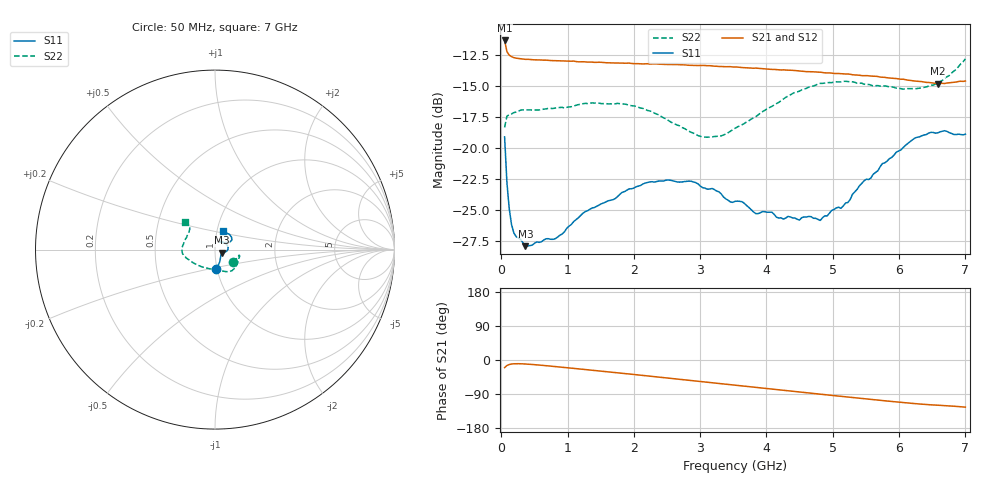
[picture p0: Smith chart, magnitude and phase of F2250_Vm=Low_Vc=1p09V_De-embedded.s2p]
! Integrated Device Technology
! Corporate Headquarters
! 6024 Silver Creek Valley Road
! San Jose, CA 95138  USA
! Phone:  1-408-284-8200
! Toll Free:  1-800-223-1366
! Webpage:  http://www.idt.com/
! Timing and RF Division
! 515 Groton Road, Suite 102
! Westford, MA 01886-6024
! Device:  F2250
! Description: Voltage Variable RF Attenuator
! Frequency:  50.0 -  6000.00 MHz
! Package:  3x3 mm Thin QFN Plastic Package: 16 pin
! Ports:  2 RF, 3 DC
!  Pin  1  = GND
!  Pin  2  = NC
!  Pin  3  = RF1  = Port 1
!  Pin  4  = NC
!  Pin  5  = GND
!  Pin  6  = GND
!  Pin  7  = GND
!  Pin  8  = GND
!  Pin  9  = NC
!  Pin 10  = RF2  = Port 2
!  Pin 11  = NC
!  Pin 12  = GND
!  Pin 13  = GND
!  Pin 14  = VCNTRL
!  Pin 15  = VDD
!  Pin 16  = VMODE
! Vcntrl:  1.090 Volts
! Vmode:  +0.000 Volts
! Vdd:  +3.30  Volts
! Current:  1.191 mA
! Data:  The device was measured on a the F2250 evaluation board which has
!  individual transmission lines to the RF pins.  Data was collected
!  using a calibrated network analyzer.  The evaluation board was
!  de-embedded using a TRL calibration technique.
!  The reference plane is the edge of the package pin.
! Misc:  SN 10
!  Action Tracker AT0258
! Date Measured:  2014-11-26
! Date:  2015-10-15  MJV
! Note:
!  Integrated Device Technology supplies this data as a sample of measured
!  data at the package pin for this product.  Your particular data for this
!  product may vary.
!  Data was taken at 25 degrees C.
!  Integrated Device Technology reserves the right to change this data at anytime.
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# GHz S dB R 50
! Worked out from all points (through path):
!   201 points, 50 MHz to 7 GHz, reference 50 ohm
!   highest |S21| = -11.34 dB at 50 MHz (marker M1); lowest = -14.8 dB at 6.583 GHz (marker M2)
!   group delay of S21, straight-line fit = 49.2 ps
!   lowest |S11| = -27.9 dB at 362.8 MHz (marker M3), VSWR 1.08, Z = 53.7 - j1.84 ohm
!   |S11| at or under -10 dB: start of sweep to end of sweep
!   |S22| runs from -19.1 to -12.8 dB; largest |S21 - S12| = 0.00084
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0.05  -19.12 -85.7  -11.34 -20.1  -11.34 -20.1  -18.35 -35.2
0.08475  -22.79 -68.4  -12.24 -14.5  -12.23 -14.5  -17.45 -19.4
0.1195  -24.90 -58.6  -12.53 -11.9  -12.51 -11.9  -17.33 -14.8
0.15425  -26.18 -50.8  -12.64 -10.6  -12.65 -10.6  -17.26 -13.4
0.22375  -27.16 -37.6  -12.77 -9.8  -12.77 -9.8  -17.12 -13.4
0.36275  -27.93 -25.2  -12.86 -10.5  -12.86 -10.5  -16.96 -14.8
0.8145  -27.33 -17.2  -12.96 -17.3  -12.98 -17.3  -16.79 -28.1
1.2315  -25.28 -16.0  -13.06 -24.6  -13.04 -24.6  -16.44 -39.2
1.857  -23.54 -6.0  -13.18 -35.7  -13.16 -35.7  -16.47 -52.2
2.37825  -22.67 5.1  -13.26 -45.1  -13.27 -45.1  -17.34 -64.5
2.86475  -22.69 19.3  -13.35 -54.1  -13.34 -54.1  -18.75 -84.9
3.0385  -23.22 24.9  -13.35 -57.3  -13.36 -57.4  -19.12 -95.1
3.3165  -23.71 35.4  -13.44 -62.5  -13.44 -62.5  -19.03 -113.3
3.525  -24.32 41.2  -13.48 -66.4  -13.49 -66.4  -18.43 -126.2
3.83775  -25.31 53.2  -13.57 -72.2  -13.57 -72.2  -17.49 -142.2
4.7065  -25.68 58.5  -13.87 -88.3  -13.87 -88.3  -15.01 -170.4
4.81075  -25.86 54.1  -13.90 -90.2  -13.89 -90.2  -14.80 -172.3
5.1235  -24.88 44.1  -14.02 -95.9  -14.03 -95.9  -14.68 -179.4
5.85325  -20.88 27.5  -14.37 -108.8  -14.36 -108.8  -15.08 163.2
6.2355  -19.22 30.6  -14.61 -114.9  -14.61 -115.0  -15.23 150.5
6.583  -18.79 40.9  -14.82 -119.3  -14.80 -119.4  -14.71 140.1
7  -18.90 66.8  -14.61 -124.3  -14.60 -124.4  -12.82 137.7
